|Texas Instruments Incorporated
| 12-Ch 7 Simultaneous Sampling, Analog Motor Control Front End w/3 1MSPS,
| 12-Bit ADCs
| Marketing part#   Digital Voltage Range   Package-type   #pins
| ADS7869IPZT   2.7V - 5.5V   TQFP   100
| ADS7869IPZTG4   2.7V - 5.5V   TQFP   100
| ADS7869IPZTR   2.7V - 5.5V   TQFP   100
| ADS7869IPZTRG4   2.7V - 5.5V   TQFP   100
[IBIS Ver]   3.2
[File name]   ads7869.ibs
|SIMDE Ver   V2.2 - 201009 - Build 424
[File Rev]   1.0
[Date]   9/19/2011
[Source]
| Texas Instruments Incorporated.
| Analog-eLab Design Center, HPA
| 12500 TI Blvd
| Dallas, TX -75243
| e-mail: elab_scm_ibis@list.ti.com
[Notes]   Revision History:
| Rev 1.0: 9/19/2011
| - Initial version of the model
| - Model generated from simulations in SPECTRE
| - Model matched to SPICE simulation
| - C_comp although listed in numerical order of value are
|   obtained from varying PVT conditions. For PVT conditions for
|   each specific value refer the buffer description under
|   respective [Model]. IBIS model user is responsible for using
|   appropriate C_comp to simulate for Signal Integrity.
| - Model names with a trailing _3p3 contains the model for
|   3.3V [3.0V and 3.6V]. Model names with a trailing _5 contains
|   the model for 5.0V [4.5V and 5.5V].
[Disclaimer]
| This model is designed as an aid for customers of Texas Instruments.
| TI and its licensors and suppliers make no warranties, either expressed
| or implied, with respect to this  model, including the warranties of
| merchantability or fitness for a particular purpose. The model is
| provided solely on an "as is" basis. The entire risk as to its quality
| and performance is with the customer.
[Copyright]
 (C) Copyright 2011 Texas Instruments Incorporated.All rights reserved.
|   ADS7869
[Component]   ADS7869
[Manufacturer]   TI
[Package]   |100 TQFP   -  PZT package
|   typ   min   max
R_pkg   0.15391   0.14355   0.17994
L_pkg   5.11494nH   4.57366nH   6.08399nH
C_pkg   0.92546pF   0.80580pF   1.10075pF
[Pin]  signal_name   model_name   R_pin   L_pin   C_pin
1   A1n   TERM   0.17150   5.86767nH  0.94706pF
2   A1p   TERM   0.16595   5.65032nH  1.05160pF
3   IUn   TERM   0.16036   5.45422nH  1.03511pF
4   IUp   TERM   0.15564   5.28381nH  1.01767pF
5   AGND   GND   0.08598   4.71585nH  1.04005pF
6   AXn   TERM   0.15503   5.14554nH  0.89754pF
7   AXp   TERM   0.15189   5.02841nH  0.87740pF
8   AVDD   POWER   0.08487   4.49117nH  0.91312pF
9   AN3n   TERM   0.15190   4.92365nH  0.84573pF
10   AN3p   TERM   0.14957   4.83522nH  0.83524pF
11   AN2n   TERM   0.14769   4.76541nH  0.82142pF
12   AN2p   TERM   0.14692   4.73456nH  0.81037pF
13   SGND   GND   0.14425   4.57936nH  0.80114pF
14   AN1n   TERM   0.14523   4.70099nH  0.80775pF
15   AN1p   TERM   0.14437   4.69986nH  0.81602pF
16   IWn   TERM   0.14461   4.73650nH  0.82743pF
17   IWp   TERM   0.14535   4.79354nH  0.83797pF
18   AVDD   POWER   0.14641   4.86540nH  0.85035pF
19   BXp   TERM   0.14778   4.94788nH  0.86858pF
20   BXn   TERM   0.15009   5.04852nH  0.88752pF
21   AGND   GND   0.15064   5.12814nH  0.97156pF
22   IVp   TERM   0.15375   5.24790nH  1.01188pF
23   IVn   TERM   0.15820   5.41306nH  1.03087pF
24   B1p   TERM   0.16356   5.60680nH  1.04676pF
25   B1n   TERM   0.16996   5.86917nH  0.93008pF
26   B2p   TERM   0.17014   5.87949nH  0.93484pF
27   B2n   TERM   0.16370   5.61537nH  1.05630pF
28   AVDD   POWER   0.15890   5.43575nH  1.03862pF
29   DAOUT   TERM   0.15502   5.28480nH  1.02360pF
30   DAIN   TERM   0.15115   5.15144nH  0.98664pF
31   U_Cp   TERM   0.14973   5.04146nH  0.90382pF
32   U_Cn   TERM   0.14740   4.94174nH  0.88452pF
33   V_Cp   TERM   0.14569   4.85304nH  0.86717pF
34   V_Cn   TERM   0.14453   4.78020nH  0.85255pF
35   W_Cp   TERM   0.14394   4.72688nH  0.84048pF
36   W_Cn   TERM   0.14382   4.69297nH  0.82725pF
37   AGND   GND   0.14466   4.69215nH  0.81575pF
38   B1   DAV_A_B   0.14355   4.57366nH  0.80580pF
39   CNTA2   INPUT   0.14551   4.70916nH  0.81734pF
40   B2   DAV_A_B   0.14573   4.73214nH  0.82679pF
41   CNTB2   INPUT   0.14658   4.78093nH  0.83999pF
42   U_COMP   OUTPUT   0.14793   4.84961nH  0.85445pF
43   V_COMP   OUTPUT   0.14961   4.93303nH  0.87058pF
44   W_COMP   OUTPUT   0.15168   5.02904nH  0.88895pF
45   U_ILIM   OUTPUT   0.15414   5.13146nH  0.90920pF
46   V_ILIM   OUTPUT   0.15557   5.24501nH  0.99178pF
47   W_ILIM   OUTPUT   0.15921   5.37422nH  1.02896pF
48   BVDD   POWER   0.16266   5.51718nH  1.04324pF
49   INT   OUTPUT   0.16657   5.67903nH  1.05820pF
50   BGND   GND   0.17138   5.91166nH  0.93170pF
51   ADDR5   ADDR   0.17994   6.08399nH  0.94886pF
52   ADDR4   ADDR   0.17282   5.80373nH  1.07810pF
53   ADDR3   ADDR   0.16679   5.59894nH  1.06017pF
54   ADDR2   ADDR   0.16158   5.42094nH  1.04104pF
55   ADDR1   ADDR   0.15710   5.27470nH  1.00104pF
56   ADDR0   ADDR   0.15489   5.14239nH  0.91844pF
57   _CS   ADDR   0.15190   5.02868nH  0.89692pF
58   _WR   ADDR   0.14964   4.92873nH  0.87756pF
59   _RD   ADDR   0.14787   4.84348nH  0.86111pF
60   DATA15   DATA   0.14662   4.77609nH  0.84804pF
61   DATA14   DATA   0.14575   4.72684nH  0.83540pF
62   DATA13   DATA   0.14579   4.70883nH  0.82655pF
63   DATA12   DATA   0.14426   4.58344nH  0.81613pF
64   DATA11   DATA   0.14583   4.70914nH  0.82622pF
65   DATA10   DATA   0.14583   4.72738nH  0.83540pF
66   DATA9   DATA   0.14675   4.77671nH  0.84840pF
67   DATA8   DATA   0.14810   4.84489nH  0.86155pF
68   DATA7   DATA   0.14984   4.92892nH  0.87761pF
69   DATA6   DATA   0.15213   5.02905nH  0.89644pF
70   DATA5   DATA   0.15496   5.13906nH  0.91680pF
71   DATA4   DATA   0.15693   5.26538nH  0.99883pF
72   DATA3   DATA   0.16099   5.40275nH  1.03792pF
73   DATA2   DATA   0.16585   5.57277nH  1.05663pF
74   DATA1   DATA   0.17148   5.76905nH  1.07390pF
75   DATA0   DATA   0.17815   6.03923nH  0.94553pF
76   BGND   GND   0.17221   5.92856nH  0.95306pF
77   CLK   INPUT   0.16625   5.66681nH  1.10075pF
78   BVDD   POWER   0.16149   5.49145nH  1.08357pF
79   _RST   INPUT   0.15752   5.34308nH  1.06535pF
80   M1   INPUT   0.15400   5.21501nH  1.03305pF
81   M0   INPUT   0.15158   5.04914nH  0.96283pF
82   AGND   GND   0.14990   4.96077nH  0.94007pF
83   DAV   DAV_A_B   0.14895   4.88792nH  0.91641pF
84   NC   NC   0.01973   2.56887nH  0.75842pF
85   AVDD   POWER   0.14572   4.73352nH  0.88864pF
86   _HOLD2   INPUT   0.14536   4.69492nH  0.88557pF
87   _HOLD1   INPUT   0.14545   4.67371nH  0.88094pF
88   CNTB1   INPUT   0.14475   4.57580nH  0.86412pF
89   A2   DAV_A_B   0.14593   4.68351nH  0.87599pF
90   CNTA1   INPUT   0.14601   4.70781nH  0.88185pF
91   A1   DAV_A_B   0.14657   4.75072nH  0.88258pF
92   NC   NC   0.01974   2.56925nH  0.75843pF
93   NC   NC   0.01996   2.62196nH  0.77284pF
94   NC   NC   0.02021   2.68050nH  0.78868pF
95   AGND   GND   0.15411   5.10082nH  0.95021pF
96   REFOUT   TERM   0.15624   5.26109nH  1.03311pF
97   REFIN   TERM   0.16006   5.39481nH  1.06728pF
98   AVDD   POWER   0.16378   5.53766nH  1.07931pF
99   A2n   TERM   0.16490   5.63889nH  1.09418pF
100   A2p   TERM   0.17075   5.88422nH  0.96083pF
|   Model Selectors
[Model Selector] INPUT
input_3p3  3.3V digital input
input_5  5.0V digital input
[Model Selector] ADDR
addr_3p3  3.3V digital input
addr_5  5.0V digital input
[Model Selector] OUTPUT
output_3p3  3.3V digital output
output_5  5.0V digital output
[Model Selector] DAV_A_B
dav_a_b_3p3  3.3V digital output
dav_a_b_5  5.0V digital output
[Model Selector] DATA
data_3p3  3.3V digital I/O
data_5  5.0V digital I/O
[Model Selector] TERM
term_3-3V  3.3V nominal termination
term_5-0V  5.0V nominal termination
[Model] term_3-3V
Model_type Terminator
C_comp   1.0e-20F  1.0e-20F  1.0e-20F
|   typ   min   max
[Voltage Range]   3.3V   3.0V   3.6V
[POWER Clamp Reference]   3.3V   3.0V   3.6V
[GND Clamp Reference]   0V   0V   0V
|Ambient Temperature   25   85   -40
|Junction Temperature
[Temperature Range]   36   96   -40
[Model] term_5-0V
Model_type Terminator
C_comp   1.0e-20F  1.0e-20F  1.0e-20F
|   typ   min   max
[Voltage Range]   5.0V   4.5V   5.5V
[POWER Clamp Reference]   5.0V   4.5V   5.5V
[GND Clamp Reference]   0V   0V   0V
|Ambient Temperature   25   85   -40
|Junction Temperature
[Temperature Range]   36   96   -40
| Models and submodels in the file (12): input_3p3 (Input), input_5 (Input), addr_3p3 (Input), addr_5 (Input), output_3p3 (Output), output_5 (Output), dav_a_b_3p3 (Output), dav_a_b_5 (Output), data_3p3 (I/O), data_5 (I/O), term_3-3V (Terminator), term_5-0V (Terminator)
